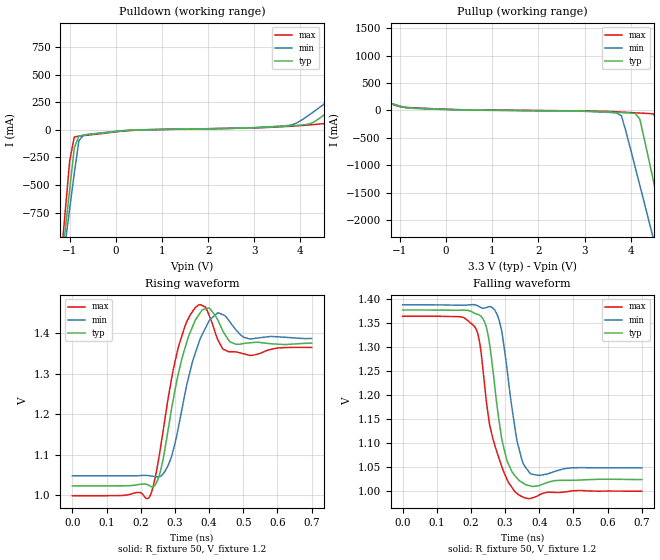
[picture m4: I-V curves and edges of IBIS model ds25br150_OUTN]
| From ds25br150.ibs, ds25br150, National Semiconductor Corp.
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[Model]   ds25br150_OUTN
Model_type Output
Polarity Inverting
Vref=1.2
Vmeas=1.2
Rref=50   | 100 Ohms Across Outputs OUTP and OUTN
Cref=0p
C_comp   1.2pF   1.2pF   1.2pF
[Temperature Range]   25   85   -40
[Voltage Range]   3.3   3.0   3.6
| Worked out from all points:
|   slope of the pulldown table from 0 to 0.495 V, typ, clamps not added: 33.5 ohm
|   slope of the pullup table from 0 to 0.495 V, typ, clamps not added: 46.1 ohm
|   rising waveform, R_fixture 50, V_fixture 1.2: 20-80 % time 45.1ps typ, 51.9ps min, 42.2ps max; typ from 1.02 V to 1.38 V
|   falling waveform, R_fixture 50, V_fixture 1.2: 20-80 % time 40.2ps typ, 39.2ps min, 50.8ps max; typ from 1.38 V to 1.02 V
[Pullup]
|Vtable   I(typ)   I(min)   I(max)
-3.6V     1.45A      1.412A     1.503A
-2.8V     789.8mA    836.5mA    773.5mA
-2.3V     519.4mA    504.5mA    549.7mA
-1V       73.28mA    80.24mA    66.81mA
3.7V      -35.52mA   -46.12mA   -25.36mA
3.8V      -39.85mA   -98.54mA   -30.02mA
4.2V      -164mA     -1.372A    -48.47mA
4.5V      -1.311A    -2.365A    -64.99mA
4.6V      -1.7A      -2.697A    -282.8mA
4.7V      -2.089A    -3.03A     -757mA
5V        -3.265A    -4.03A     -2.204A
7.2V      -11.88A    -11.34A    -12.91A
[Pulldown]
|V(pulldown)   I(typ)   I(min)   I(max)
-3.6V     -10.72A    -9.365A    -12.93A
-1.2V     -1.31A     -1.371A    -1.236A
-1.1V     -923.5mA   -1.042A    -755.8mA
-1V       -539.7mA   -715.6mA   -281.7mA
-900mV    -163.9mA   -392.5mA   -64.37mA
-800mV    -55.71mA   -99.4mA    -56.83mA
3.8V      36.73mA    43.96mA    32.98mA
4.6V      164mA      262.4mA    66.5mA
5.3V      411.1mA    511.7mA    312.3mA
5.9V      657mA      919.7mA    557.5mA
6.4V      1.051A     1.282A     785mA
7.2V      1.718A     1.864A     1.522A
[Ramp]
|   typ   min   max
dV/dt_r   212m/36p   201m/43p   219m/37p
dV/dt_f   212m/36p   201m/43p   219m/37p
R_load=50
[Rising Waveform]
R_fixture=50
V_fixture=1.2
V_fixture_min=1.218
V_fixture_max=1.1817
0s        1.023V     1.048V     999.1mV
225ps     1.024V     1.048V     995.7mV
255ps     1.052V     1.046V     1.102V
290ps     1.213V     1.095V     1.287V
330ps     1.364V     1.253V     1.418V
370ps     1.444V     1.376V     1.469V
400ps     1.462V     1.43V      1.443V
455ps     1.385V     1.434V     1.354V
520ps     1.376V     1.385V     1.344V
700ps     1.375V     1.386V     1.364V
[Falling Waveform]
R_fixture=50
V_fixture=1.2
V_fixture_min=1.218
V_fixture_max=1.1817
0s        1.377V     1.388V     1.364V
180ps     1.377V     1.387V     1.361V
220ps     1.368V     1.386V     1.328V
235ps     1.359V     1.381V     1.255V
255ps     1.304V     1.385V     1.137V
285ps     1.134V     1.349V     1.062V
305ps     1.064V     1.258V     1.025V
335ps     1.027V     1.104V     994.7mV
375ps     1.01V      1.036V     984.6mV
700ps     1.024V     1.048V     999.5mV
